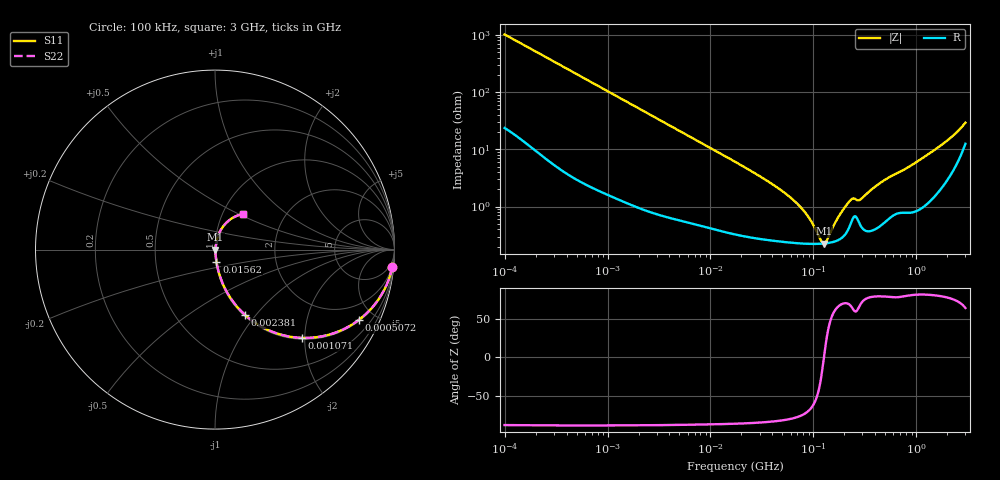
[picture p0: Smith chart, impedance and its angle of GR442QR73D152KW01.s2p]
!Murata Part Number: GR442QR73D152KW01
!These Parameters are Measured in Series Mode Connection
!Data Generated on Mar 13, 2026
!  o--ll--o
!Port1  Port2
!  o------o
!Operation Temp=25[degC], DC Bias Voltage=0[V]
!Freq. Start=100[kHz] Stop=3[GHz] 401[Steps]
# Hz S RI R 50
!Freq.(Hz) S11(Real) S11(Imag) S21(Real) S21(Imag) S12(Real) S12(Imag) S22(Real) S22(Imag)
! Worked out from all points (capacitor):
!   401 points, 100 kHz to 3 GHz, reference 50 ohm
!   read as one part in series: C = 1.56 nF near 105.3 kHz
!   lowest |Z| = 226 mohm at 126 MHz (marker M1)
!   series resonance near 126.7 MHz, so ESL is about 1 nH
!   S11 on the Smith chart (normalised r, x): 100 kHz: 1, -20; 507.2 kHz: 1.06, -4.08; 1.071 MHz: 1.03, -1.94; 2.381 MHz: 1.02, -0.88; 15.62 MHz: 1.01, -0.13; 3 GHz: 1.25, +0.53
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100000  0.9882 -0.097  0.0118 0.097  0.0118 0.097  0.9882 -0.097
259498  0.937 -0.235  0.063 0.235  0.063 0.235  0.937 -0.235
507162  0.8029 -0.3908  0.1971 0.3908  0.1971 0.3908  0.8029 -0.3908
562235  0.769 -0.4144  0.231 0.4144  0.231 0.4144  0.769 -0.4144
1070873  0.4855 -0.492  0.5145 0.492  0.5145 0.492  0.4855 -0.492
2380755  0.1666 -0.3631  0.8334 0.3631  0.8334 0.3631  0.1666 -0.3631
3161081  0.1042 -0.2949  0.8958 0.2949  0.8958 0.2949  0.1042 -0.2949
6674626  0.029 -0.1526  0.971 0.1526  0.971 0.1526  0.029 -0.1526
1.56239e7  0.00788 -0.0667  0.9921 0.0667  0.9921 0.0667  0.00788 -0.0667
1.77727e7  0.00667 -0.0586  0.9933 0.0586  0.9933 0.0586  0.00667 -0.0586
5.667996e7  0.0026 -0.0154  0.9974 0.0154  0.9974 0.0154  0.0026 -0.0154
7.722238e7  0.00234 -0.00895  0.9977 0.00895  0.9977 0.00895  0.00234 -0.00895
9.738194e7  0.00225 -0.00466  0.9978 0.00466  0.9978 0.00466  0.00225 -0.00466
1.166348e8  0.00224 -0.00147  0.9978 0.00147  0.9978 0.00147  0.00224 -0.00147
1.260104e8  0.00226 -0.000101  0.9977 0.000101  0.9977 0.000101  0.00226 -0.000101
1.361397e8  0.00229 0.00128  0.9977 -0.00128  0.9977 -0.00128  0.00229 0.00128
1.807614e8  0.00273 0.00668  0.9973 -0.00668  0.9973 -0.00668  0.00273 0.00668
2.279507e8  0.00487 0.0118  0.9951 -0.0118  0.9951 -0.0118  0.00487 0.0118
2.874592e8  0.00479 0.0124  0.9952 -0.0124  0.9952 -0.0124  0.00479 0.0124
5.475153e8  0.00718 0.0317  0.9928 -0.0317  0.9928 -0.0317  0.00718 0.0317
1.7917e9  0.0349 0.1138  0.9651 -0.1138  0.9651 -0.1138  0.0349 0.1138
3e9  0.1575 0.1974  0.8425 -0.1974  0.8425 -0.1974  0.1575 0.1974
